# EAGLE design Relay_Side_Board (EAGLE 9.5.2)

## Sheet 1 of 2: Relay side expansion board for hoop house controller - main controller section
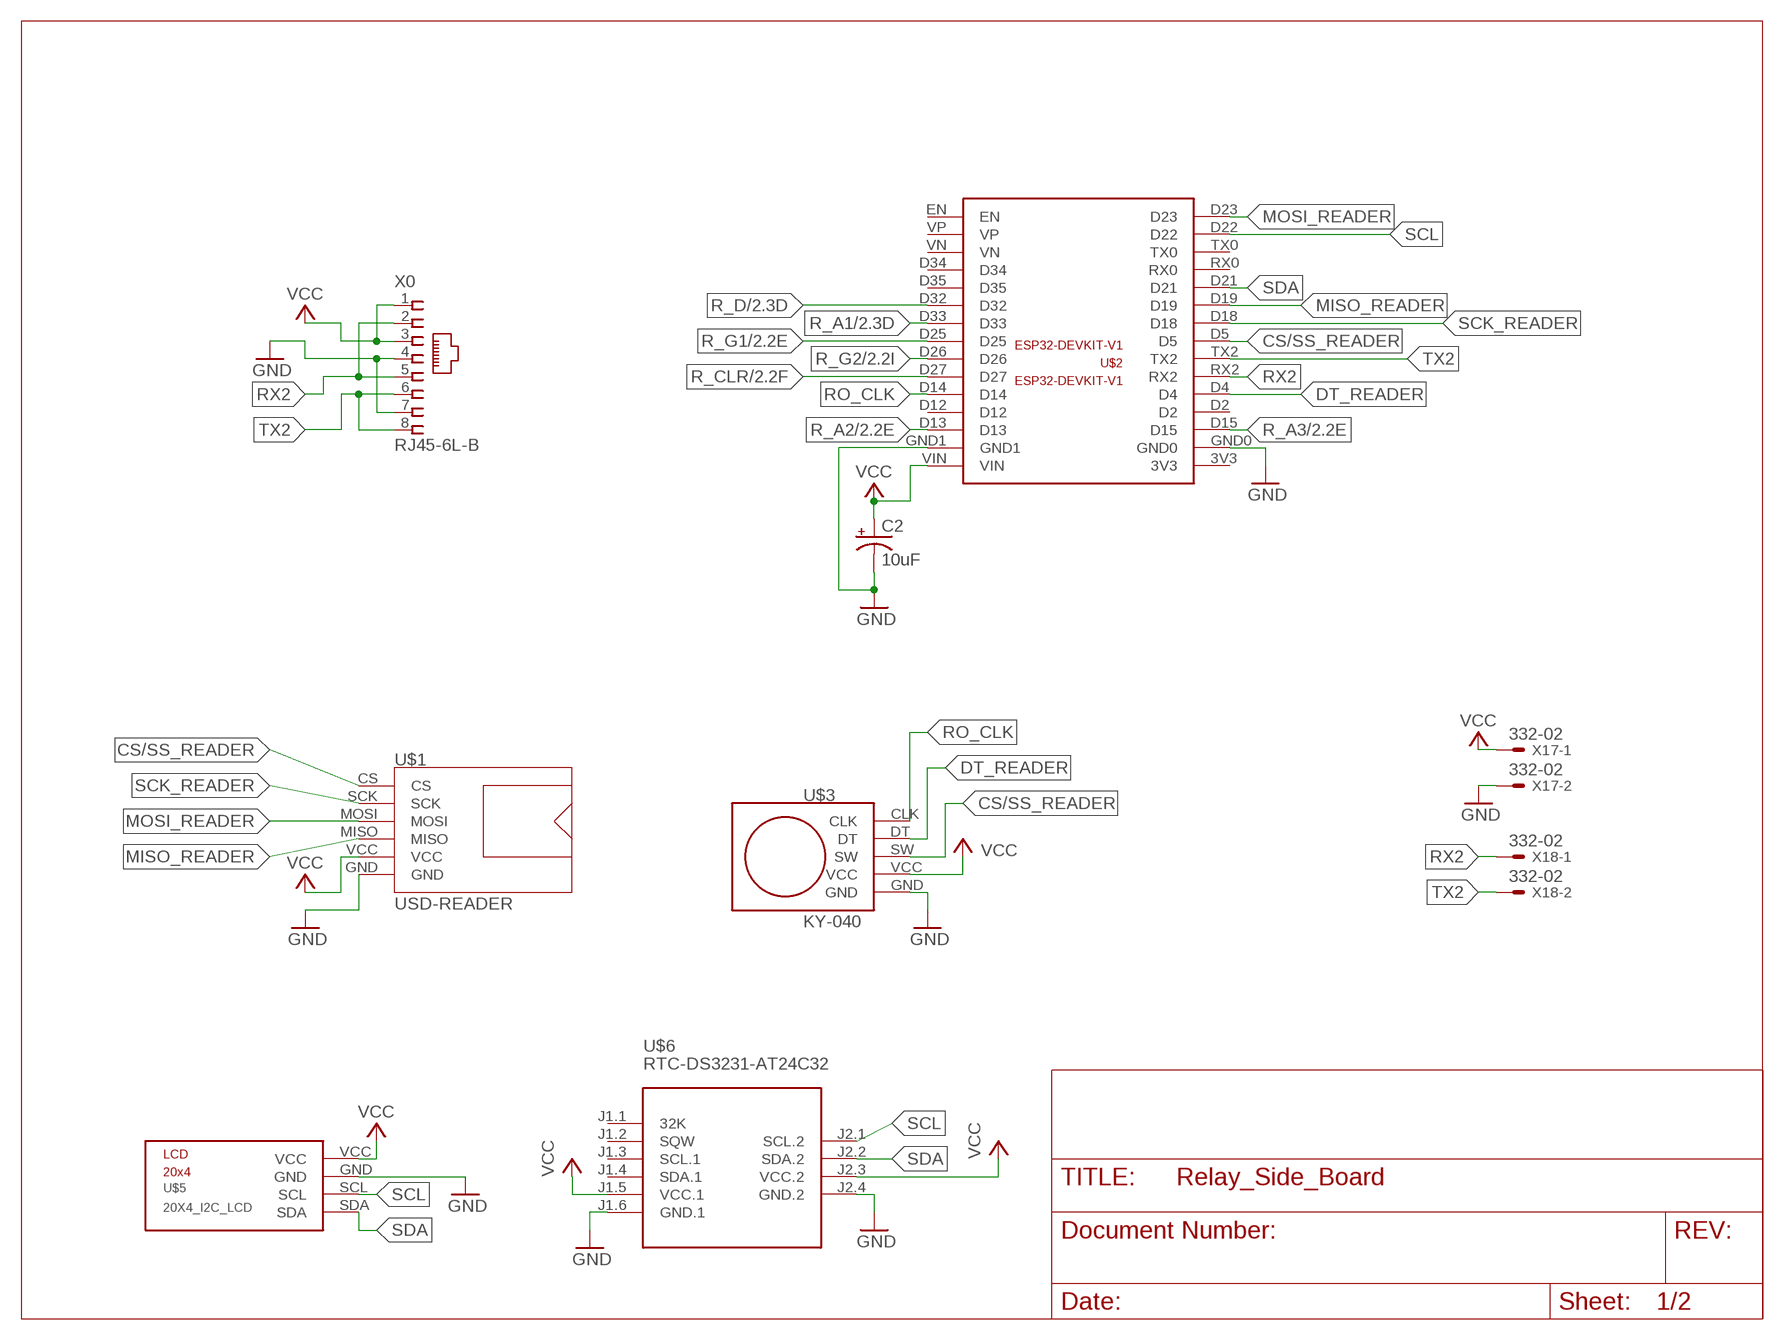
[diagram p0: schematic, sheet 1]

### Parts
C2  10uF  CPOL-USE3.5-10  [E3,5-10]
U$1  USD-READER  [USD-READER]
U$2  ESP32-DEVKIT-V1  [ESP32-DEVKIT-V1]
U$3  KY-040  [ROTARY-ENCODER]
U$5  20X4_I2C_LCD  [I2C_LCD]
U$6  RTC-DS3231-AT24C32  [RTC-DS3231-AT24C32]
X0  RJ45-6L-B  [RJ45-NO-SHIELD]
X17  332-02  [332-02]
X18  332-02  [332-02]

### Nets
CS/SS_READER: U$1.CS U$2.D5 U$3.SW
DT_READER: U$2.D4 U$3.DT
GND: C2.- U$1.GND U$2.GND0 U$2.GND1 U$3.GND U$5.GND U$6.J1.6(GND.1) U$6.J2.4(GND.2) X0.4 X0.7 X17.2 ; also sheet 2
MISO_READER: U$1.MISO U$2.D19
MOSI_READER: U$1.MOSI U$2.D23
R_A1: U$2.D33 ; also sheet 2
R_A2: U$2.D13 ; also sheet 2
R_A3: U$2.D15 ; also sheet 2
R_CLR: U$2.D27 ; also sheet 2
R_D: U$2.D32 ; also sheet 2
R_G1: U$2.D25 ; also sheet 2
R_G2: U$2.D26 ; also sheet 2
RO_CLK: U$2.D14 U$3.CLK
RX2: U$2.RX2 X0.2 X0.5 X18.1
SCK_READER: U$1.SCK U$2.D18
SCL: U$2.D22 U$5.SCL U$6.J2.1(SCL.2)
SDA: U$2.D21 U$5.SDA U$6.J2.2(SDA.2)
TX2: U$2.TX2 X0.6 X0.8 X18.2
VCC: C2.+ U$1.VCC U$2.VIN U$3.VCC U$5.VCC U$6.J1.5(VCC.1) U$6.J2.3(VCC.2) X0.1 X0.3 X17.1 ; also sheet 2
Unconnected: U$2.3V3 U$2.D2 U$2.D12 U$2.D34 U$2.D35 U$2.EN U$2.RX0 U$2.TX0 U$2.VN U$2.VP U$6.J1.1(32K) U$6.J1.2(SQW) U$6.J1.3(SCL.1) U$6.J1.4(SDA.1)

## Sheet 2 of 2: Relay side expansion board for hoop house controller - addressed relays with memory
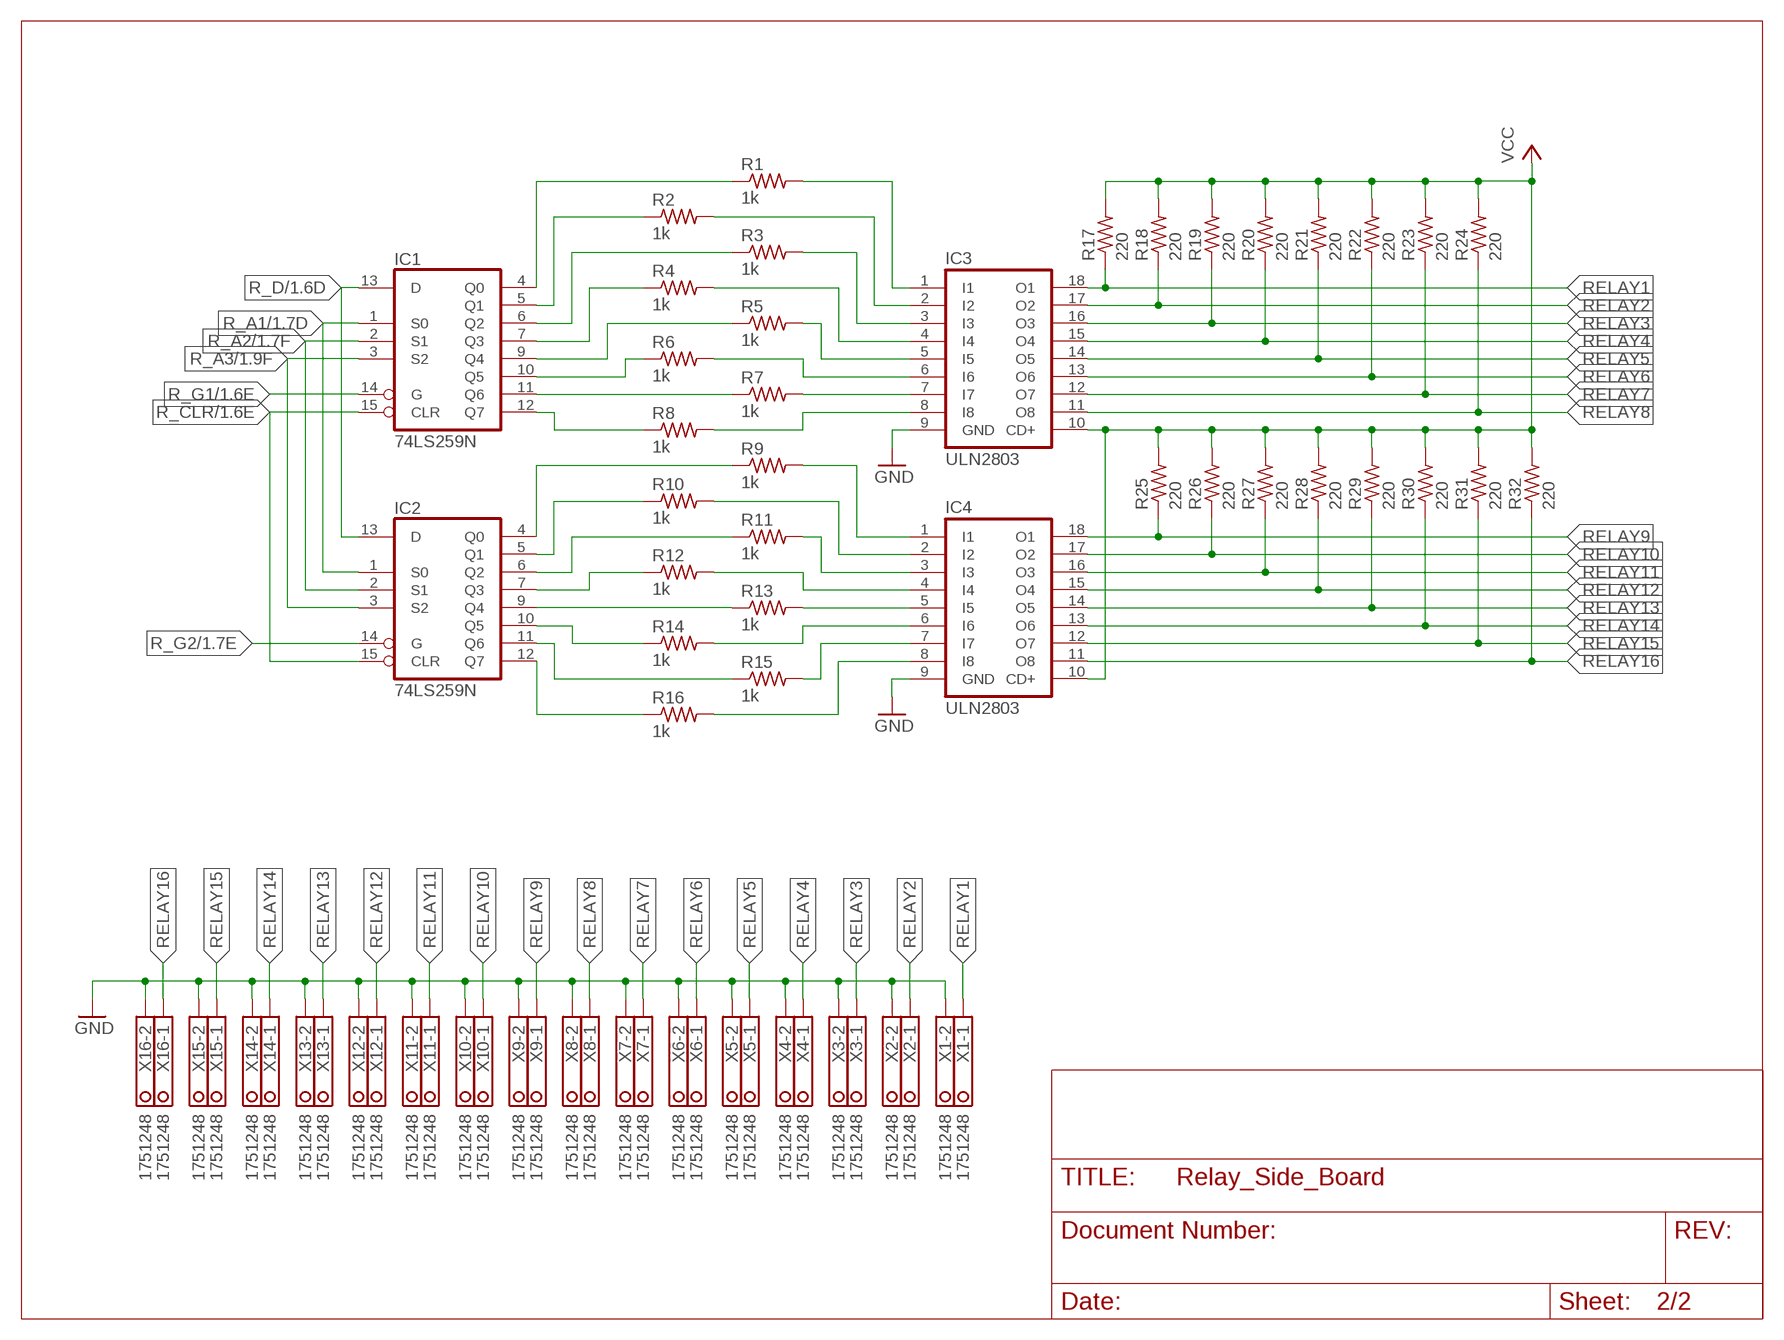
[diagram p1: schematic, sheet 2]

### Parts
IC1  74LS259N  [DIL16]
IC2  74LS259N  [DIL16]
IC3  ULN2803  ULN2803A  [DIL18]
IC4  ULN2803  ULN2803A  [DIL18]
R1  1k  R-US_R0805  [R0805]
R2  1k  R-US_R0805  [R0805]
R3  1k  R-US_R0805  [R0805]
R4  1k  R-US_R0805  [R0805]
R5  1k  R-US_R0805  [R0805]
R6  1k  R-US_R0805  [R0805]
R7  1k  R-US_R0805  [R0805]
R8  1k  R-US_R0805  [R0805]
R9  1k  R-US_R0805  [R0805]
R10  1k  R-US_R0805  [R0805]
R11  1k  R-US_R0805  [R0805]
R12  1k  R-US_R0805  [R0805]
R13  1k  R-US_R0805  [R0805]
R14  1k  R-US_R0805  [R0805]
R15  1k  R-US_R0805  [R0805]
R16  1k  R-US_R0805  [R0805]
R17  220  R-US_R0805  [R0805]
R18  220  R-US_R0805  [R0805]
R19  220  R-US_R0805  [R0805]
R20  220  R-US_R0805  [R0805]
R21  220  R-US_R0805  [R0805]
R22  220  R-US_R0805  [R0805]
R23  220  R-US_R0805  [R0805]
R24  220  R-US_R0805  [R0805]
R25  220  R-US_R0805  [R0805]
R26  220  R-US_R0805  [R0805]
R27  220  R-US_R0805  [R0805]
R28  220  R-US_R0805  [R0805]
R29  220  R-US_R0805  [R0805]
R30  220  R-US_R0805  [R0805]
R31  220  R-US_R0805  [R0805]
R32  220  R-US_R0805  [R0805]
X1  1751248  [1751248]
X2  1751248  [1751248]
X3  1751248  [1751248]
X4  1751248  [1751248]
X5  1751248  [1751248]
X6  1751248  [1751248]
X7  1751248  [1751248]
X8  1751248  [1751248]
X9  1751248  [1751248]
X10  1751248  [1751248]
X11  1751248  [1751248]
X12  1751248  [1751248]
X13  1751248  [1751248]
X14  1751248  [1751248]
X15  1751248  [1751248]
X16  1751248  [1751248]

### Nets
GND: IC3.9(GND) IC4.9(GND) X1.2 X2.2 X3.2 X4.2 X5.2 X6.2 X7.2 X8.2 X9.2 X10.2 X11.2 X12.2 X13.2 X14.2 X15.2 X16.2 ; also sheet 1
N$1: IC1.4(Q0) R1.1
N$2: IC1.5(Q1) R2.1
N$3: IC1.6(Q2) R3.1
N$4: IC1.7(Q3) R4.1
N$5: IC1.9(Q4) R5.1
N$6: IC1.10(Q5) R6.1
N$7: IC1.11(Q6) R7.1
N$8: IC1.12(Q7) R8.1
N$9: IC2.4(Q0) R9.1
N$10: IC2.5(Q1) R10.1
N$11: IC2.6(Q2) R11.1
N$12: IC2.7(Q3) R12.1
N$13: IC4.5(I5) R13.2
N$14: IC2.10(Q5) R14.1
N$15: IC2.11(Q6) R15.1
N$16: IC2.12(Q7) R16.1
N$17: IC3.1(I1) R1.2
N$18: IC3.2(I2) R2.2
N$19: IC3.3(I3) R3.2
N$20: IC3.4(I4) R4.2
N$21: IC3.5(I5) R5.2
N$22: IC3.6(I6) R6.2
N$23: IC3.7(I7) R7.2
N$24: IC3.8(I8) R8.2
N$25: IC2.9(Q4) R13.1
N$26: IC4.6(I6) R14.2
N$49: IC4.1(I1) R9.2
N$50: IC4.2(I2) R10.2
N$51: IC4.3(I3) R11.2
N$52: IC4.4(I4) R12.2
N$55: IC4.7(I7) R15.2
N$56: IC4.8(I8) R16.2
R_A1: IC1.1(S0) IC2.1(S0) ; also sheet 1
R_A2: IC1.2(S1) IC2.2(S1) ; also sheet 1
R_A3: IC1.3(S2) IC2.3(S2) ; also sheet 1
R_CLR: IC1.15(CLR) IC2.15(CLR) ; also sheet 1
R_D: IC1.13(D) IC2.13(D) ; also sheet 1
R_G1: IC1.14(G) ; also sheet 1
R_G2: IC2.14(G) ; also sheet 1
RELAY1: IC3.18(O1) R17.1 X1.1
RELAY2: IC3.17(O2) R18.1 X2.1
RELAY3: IC3.16(O3) R19.1 X3.1
RELAY4: IC3.15(O4) R20.1 X4.1
RELAY5: IC3.14(O5) R21.1 X5.1
RELAY6: IC3.13(O6) R22.1 X6.1
RELAY7: IC3.12(O7) R23.1 X7.1
RELAY8: IC3.11(O8) R24.1 X8.1
RELAY9: IC4.18(O1) R25.1 X9.1
RELAY10: IC4.17(O2) R26.1 X10.1
RELAY11: IC4.16(O3) R27.1 X11.1
RELAY12: IC4.15(O4) R28.1 X12.1
RELAY13: IC4.14(O5) R29.1 X13.1
RELAY14: IC4.13(O6) R30.1 X14.1
RELAY15: IC4.12(O7) R31.1 X15.1
RELAY16: IC4.11(O8) R32.1 X16.1
VCC: IC3.10(CD+) IC4.10(CD+) R17.2 R18.2 R19.2 R20.2 R21.2 R22.2 R23.2 R24.2 R25.2 R26.2 R27.2 R28.2 R29.2 R30.2 R31.2 R32.2 ; also sheet 1

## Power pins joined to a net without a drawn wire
GND: IC1.8(GND) IC2.8(GND)
VCC: IC1.16(VCC) IC2.16(VCC)

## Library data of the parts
C2 = rcl:CPOL-US: POLARIZED CAPACITOR, American symbol; SPICEPREFIX: C
IC1 IC2 = 74xx-us:74*259: 8-bit addressable LATCH
IC3 IC4 = uln-udn:ULN2803A: DRIVER ARRAY
R1-R32 = rcl:R-US_: RESISTOR, American symbol; SPICEPREFIX: R
U$1 = FF Hoop House Controller:USD-READER
U$2 = FF Hoop House Controller:ESP32-DEVKIT-V1
U$3 = FF Hoop House Controller:KY-040
U$5 = FF Hoop House Controller:20X4_I2C_LCD
U$6 = diy-modules:RTC-DS3231-AT24C32: RTC Module with Battery and EEPROM based on DS3231 and AT24C32 chips Tutorial can be found here: https://edwardmallon.wordpress.com/2014/05/21/using-a-cheap-3-ds3231-rtc-at24c32-eeprom-from-ebay/ Click here to find device on ebay.com
X0 = con-tycoelectronics:RJ45: CORCOM Modular RJ Jacks No Shield Source: www.tycoelectronics.com .. ENG_DS_1654001_1099_RJ_L_0507.pdf; MPN: RJ45-6L-B; OC_FARNELL: unknown; OC_NEWARK: 16R6090
X1-X16 = con-phoenix-350:1751248: MKDS 1/ 2-3,5 Printklemme; OC_FARNELL: unknown; OC_NEWARK: unknown
X17 X18 = con-garry:332-02: 2 Pin - 2mm Dual Row

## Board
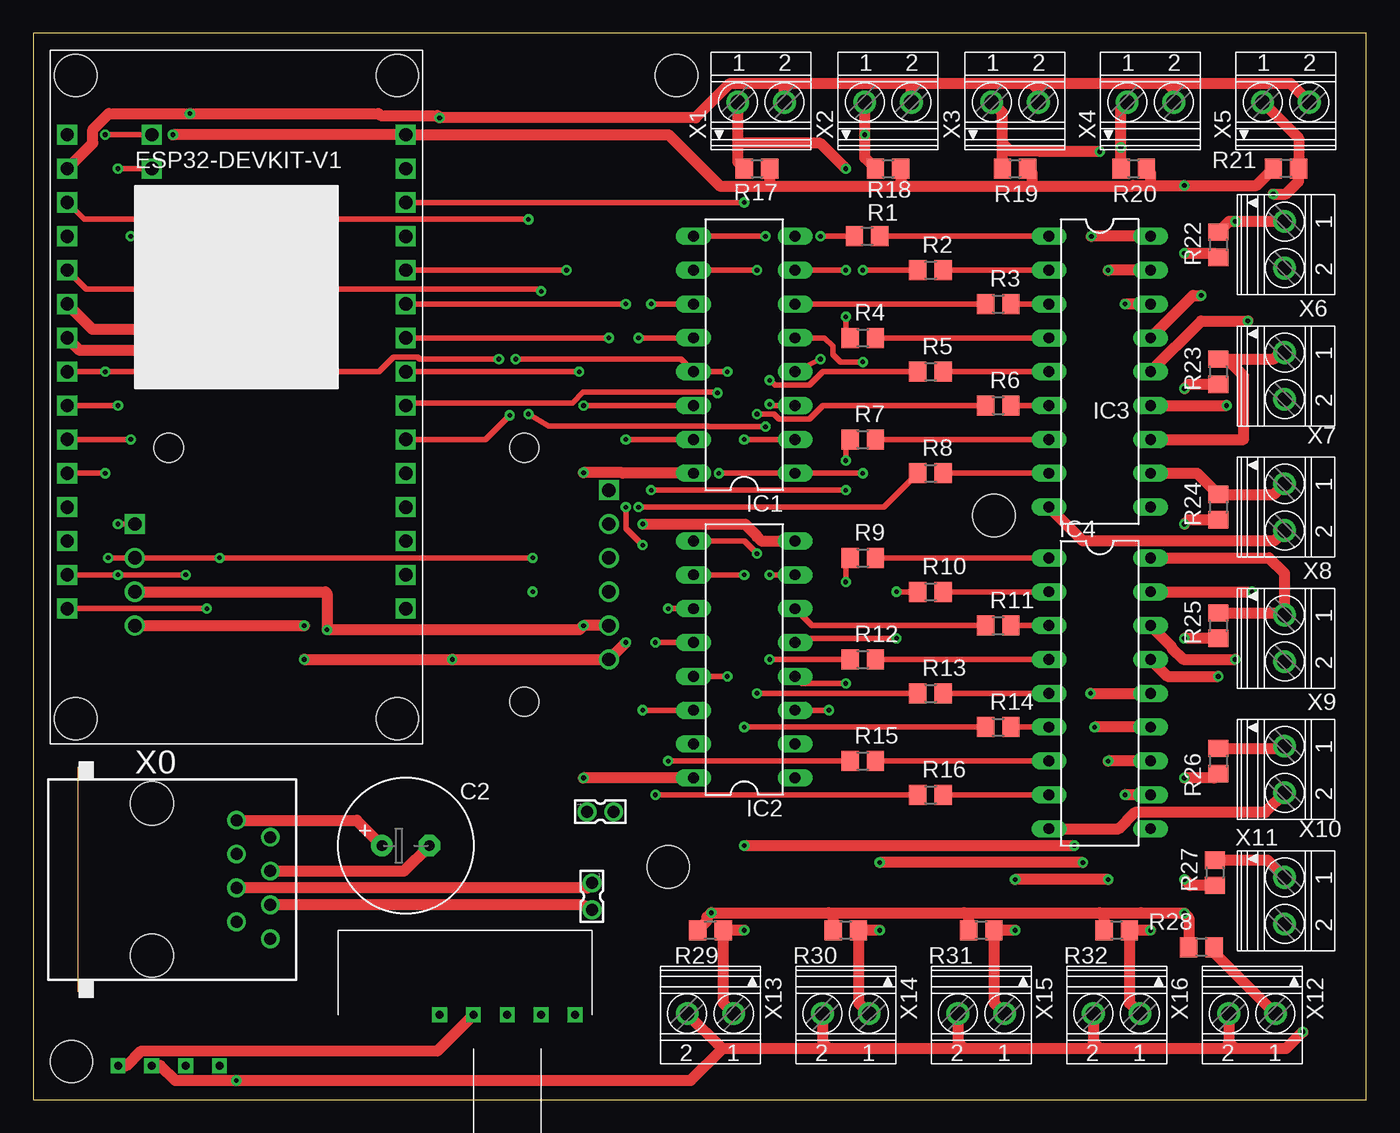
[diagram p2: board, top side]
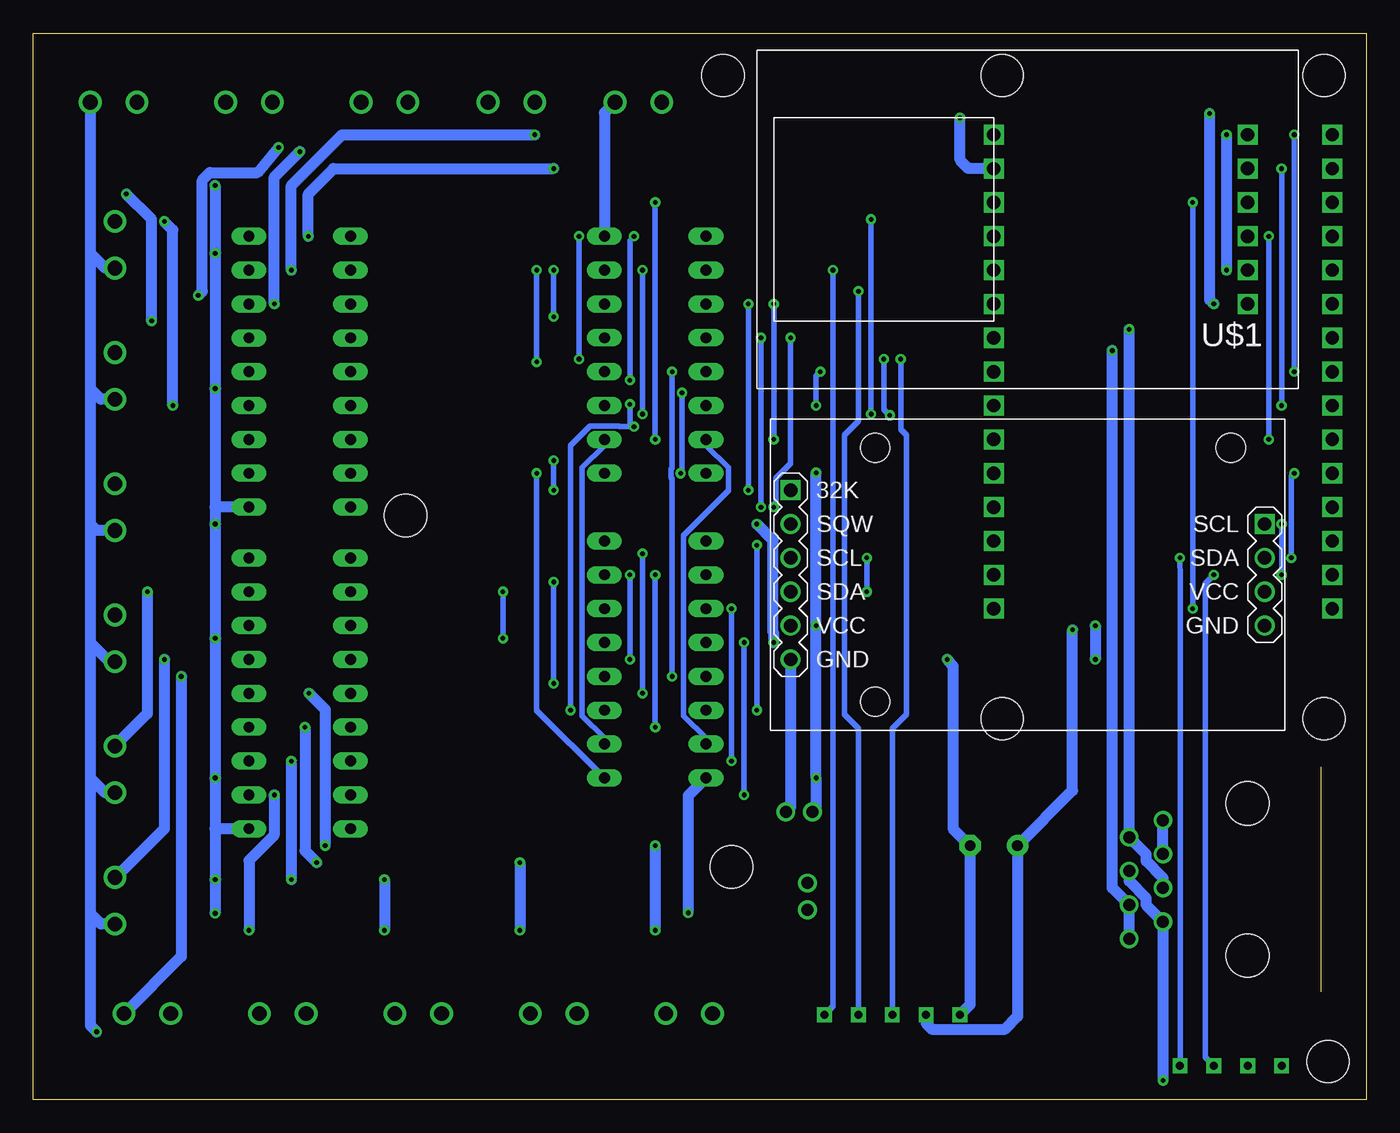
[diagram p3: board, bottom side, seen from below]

Size 100 x 80 mm. Coordinates in mm from the lower left corner, seen from the top.
Outline: 0,0 100,0 100,80 0,80 0,0
Copper layers (1*16): Top 0.035mm / dielectric 1.5mm / Bottom 0.035mm
Design rules "default": minimum track width 6mil, minimum drill 0.35mm, track to track 6mil, track to pad 6mil, pad to pad 6mil, via to via 6mil, smd to smd 6mil, copper to edge 40mil, drill to drill 6mil, minimum pad ring 10mil, minimum via ring 8mil, stop-mask expansion 4mil, vias tented up to drill 0mil, thermal gap 10mil
Holes 3.17 mm at 3.17,28.57 27.3,28.57 27.3,76.83 3.17,76.83 72.07,43.81 47.62,17.46 2.86,2.86 48.26,76.83

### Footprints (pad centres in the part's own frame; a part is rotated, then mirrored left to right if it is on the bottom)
E3,5-10 = drill 0.813 pad 1.6: + -1.778,0 | drill 0.813 pad 1.6 octagon: - 1.778,0
DIL16 = drill 0.813 long: 1 -8.89,-3.81; 2 -6.35,-3.81; 3 -3.81,-3.81; 4 -1.27,-3.81; 5 1.27,-3.81; 6 3.81,-3.81; 7 6.35,-3.81; 8 8.89,-3.81; 9 8.89,3.81; 10 6.35,3.81; 11 3.81,3.81; 12 1.27,3.81; 13 -1.27,3.81; 14 -3.81,3.81; 15 -6.35,3.81; 16 -8.89,3.81
DIL18 = drill 0.813 long: 1 -10.16,-3.81; 2 -7.62,-3.81; 3 -5.08,-3.81; 4 -2.54,-3.81; 5 0,-3.81; 6 2.54,-3.81; 7 5.08,-3.81; 8 7.62,-3.81; 9 10.16,-3.81; 10 10.16,3.81; 11 7.62,3.81; 12 5.08,3.81; 13 2.54,3.81; 14 0,3.81; 15 -2.54,3.81; 16 -5.08,3.81; 17 -7.62,3.81; 18 -10.16,3.81
R0805 = smd 1.3 x 1.5: 1 -0.95,0; 2 0.95,0
USD-READER = drill 1 square: CS -5.08,-6.35; GND -5.08,6.35; MISO -5.08,1.27; MOSI -5.08,-1.27; SCK -5.08,-3.81; VCC -5.08,3.81
ESP32-DEVKIT-V1 = drill 1 square: 3V3 -12.7,17.78; D2 -12.7,10.16; D4 -12.7,7.62; D5 -12.7,0; D12 12.7,10.16; D13 12.7,12.7; D14 12.7,7.62; D15 -12.7,12.7; D18 -12.7,-2.54; D19 -12.7,-5.08; D21 -12.7,-7.62; D22 -12.7,-15.24; D23 -12.7,-17.78; D25 12.7,0; D26 12.7,2.54; D27 12.7,5.08; D32 12.7,-5.08; D33 12.7,-2.54; D34 12.7,-10.16; D35 12.7,-7.62; EN 12.7,-17.78; GND0 -12.7,15.24; GND1 12.7,15.24; RX0 -12.7,-10.16; RX2 -12.7,5.08; TX0 -12.7,-12.7; TX2 -12.7,2.54; VIN 12.7,17.78; VN 12.7,-12.7; VP 12.7,-15.24
ROTARY-ENCODER = drill 0.6 square: CLK 0,5.08; DT 0,2.54; GND 0,-5.08; SW 0,0; VCC 0,-2.54
I2C_LCD = drill 0.6 square: GND 0,1.27; SCL 0,-1.27; SDA 0,-3.81; VCC 0,3.81
RTC-DS3231-AT24C32 = drill 1 square: J1.1 -17.78,6.35; J2.1 17.78,3.81 | drill 1: J1.2 -17.78,3.81; J1.3 -17.78,1.27; J1.4 -17.78,-1.27; J1.5 -17.78,-3.81; J1.6 -17.78,-6.35; J2.2 17.78,1.27; J2.3 17.78,-1.27; J2.4 17.78,-3.81 | hole 2.2: -11.43,-9.525; -11.43,9.525; 15.24,9.525
RJ45-NO-SHIELD = drill 0.9 pad 1.4: 1 -4.445,6.35; 2 -3.175,8.89; 3 -1.905,6.35; 4 -0.635,8.89; 5 0.635,6.35; 6 1.905,8.89; 7 3.175,6.35; 8 4.445,8.89 | hole 3.251: -5.715,0; 5.715,0
1751248 = drill 1.1 pad 1.7: 1 -1.75,-0.1; 2 1.75,-0.1
332-02 = drill 0.9 pad 1.27: 1 0,-1; 2 0,1

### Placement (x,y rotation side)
C2  27.94,19.05 0 top
IC1  53.34,55.88 90 top
IC2  53.34,33.02 90 top
IC3  80.01,54.61 270 top
IC4  80.01,30.48 270 top
R1  62.55,64.77 0 top
R2  67.31,62.23 0 top
R3  72.39,59.69 0 top
R4  62.23,57.15 0 top
R5  67.31,54.61 0 top
R6  72.39,52.07 0 top
R7  62.23,49.53 0 top
R8  67.31,46.99 0 top
R9  62.23,40.64 0 top
R10  67.31,38.1 0 top
R11  72.39,35.56 0 top
R12  62.23,33.02 0 top
R13  67.31,30.48 0 top
R14  72.39,27.94 0 top
R15  62.23,25.4 0 top
R16  67.31,22.86 0 top
R17  54.3,69.85 0 top
R18  64.14,69.85 0 top
R19  73.66,69.85 0 top
R20  82.55,69.85 0 top
R21  93.98,69.85 180 top
R22  88.9,64.14 270 top
R23  88.9,54.61 270 top
R24  88.9,44.45 270 top
R25  88.9,35.56 270 top
R26  88.9,25.4 270 top
R27  88.65,17.02 270 top
R28  87.63,11.43 180 top
R29  50.8,12.7 180 top
R30  60.96,12.7 180 top
R31  71.12,12.7 180 top
R32  81.28,12.7 180 top
U$1  13.97,66.04 180 bottom
U$2  15.24,54.61 0 top
U$3  35.56,6.35 270 top
U$5  10.16,2.54 90 top
U$6  25.4,39.37 0 bottom
X0  8.89,16.51 270 top
X1  54.61,74.93 0 top
X2  64.14,74.93 0 top
X3  73.66,74.93 0 top
X4  83.82,74.93 0 top
X5  93.98,74.93 0 top
X6  93.98,64.14 270 top
X7  93.98,54.29 270 top
X8  93.98,44.45 270 top
X9  93.98,34.61 270 top
X10  93.98,24.77 270 top
X11  93.98,14.92 270 top
X12  91.44,6.35 180 top
X13  50.8,6.35 180 top
X14  60.96,6.35 180 top
X15  71.12,6.35 180 top
X16  81.28,6.35 180 top
X17  42.55,21.59 270 top
X18  41.91,15.24 180 top

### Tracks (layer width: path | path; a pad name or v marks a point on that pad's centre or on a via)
CS/SS_READER  (via drill 0.35)
  Top 0.406: U$2.D5 v5.4,54.61 25.93,54.61 27.04,55.72 28.84,55.72 29,55.56 v34.92,55.56 | v5.4,72.39 U$1.CS
  Bottom 0.406: v5.4,72.39 v5.4,54.61 | U$3.SW 35.56,27.84 34.51,28.88 34.51,49.86 34.92,50.27 v34.92,55.56
DT_READER  (via drill 0.35)
  Top 0.406: v38.1,60.64 37.94,60.8 3.97,60.8 U$2.D4
  Bottom 0.406: v38.1,60.64 38.1,50.91 39.15,49.86 39.15,28.88 38.1,27.84 U$3.DT
GND  (via drill 0.35)
  Top 0.813: v11.43,59.69 U$1.GND | IC2.8 54.61,41.91 54.28,42.24 54.28,42.3 53.4,43.18 v45.72,43.18 | v44.45,34.29 U$6.J1.6 v31.43,33.02 v20.32,33.02 | U$6.J2.4 v20.32,35.56 | 56.52,76.24 52.28,76.24 49.7,73.66 v30.48,73.66 30.32,73.83 26.06,73.83 25.91,73.98 v11.75,73.98 5.66,73.98 4.46,72.78 4.46,71.77 U$2.GND0 | 56.52,76.24 66.04,76.24 | 66.04,76.24 74.93,76.24 | 74.93,76.24 85.09,76.24 | 85.09,76.24 94.32,76.24 X5.2 | v95.25,5.08 93.98,3.81 90.17,3.81 | 90.17,3.81 80.01,3.81 | 80.01,3.81 69.85,3.81 | 69.85,3.81 59.69,3.81 | 74.93,76.24 75.41,75.76 X3.2 | 85.09,76.24 85.57,75.76 X4.2 | 90.17,3.81 89.69,4.29 X12.2 | 80.01,3.81 79.53,4.29 X16.2 | 69.85,3.81 69.37,4.29 X15.2 | 59.69,3.81 59.21,4.29 X14.2 | 59.69,3.81 51.69,3.81 | IC3.9 78.74,41.91 93.09,41.91 X8.2 | IC4.9 81.44,20.32 82.66,21.54 92.4,21.54 X10.2 | 56.52,76.24 56.36,76.08 X1.2 | 66.04,76.24 65.89,76.08 X2.2 | U$5.GND 9.53,2.54 10.64,1.43 v15.24,1.43 49.31,1.43 51.69,3.81 | X13.2 51.69,3.81 | X0.4 27.81,17.14 C2.-
  Bottom 0.813: v11.43,59.69 11.75,60.01 v11.75,73.98 | v31.43,33.02 30.99,32.51 30.99,20.32 C2.- 29.72,7.11 U$3.GND | v44.45,34.29 44.45,34.97 44.49,35.02 44.49,41.95 v45.72,43.18 | v20.32,35.56 v20.32,33.02 | U$2.GND1 29.84,69.85 30.48,70.48 v30.48,73.66 | 95.73,63.5 95.73,53.34 | 95.73,53.34 95.73,43.18 | 95.73,43.18 95.73,34.29 | 95.73,34.29 95.73,24.13 | 95.73,24.13 95.73,13.97 | 95.73,13.97 95.73,5.56 v95.25,5.08 | 95.73,53.34 94.93,52.54 X7.2 | 95.73,43.18 95.25,42.7 X8.2 | 95.73,34.29 94.3,32.86 X9.2 | 95.73,24.13 94.61,23.02 X10.2 | 95.73,13.97 94.93,13.17 X11.2 | 95.73,63.5 94.61,62.38 X6.2 | IC1.8 57.15,74.04 X1.2 | X5.2 95.73,63.5 | X0.4 17.78,16.39 16.52,15.13 16.52,14.61 X0.7 v15.24,1.43 | U$6.J1.6 43.18,21.95 X17.2
MISO_READER  (via drill 0.35)
  Top 0.406: U$2.D19 v7.3,49.53 | v7.3,64.77 U$1.MISO
  Bottom 0.406: v7.3,49.53 v7.3,64.77
MOSI_READER  (via drill 0.35)
  Top 0.406: U$2.D23 v13.02,36.83 | v13.02,67.31 U$1.MOSI
  Bottom 0.406: v13.02,67.31 v13.02,36.83
N$1  (via drill 0.35)
  Top 0.406: IC1.4 v59.05,55.56 | R1.1 v59.05,64.77
  Bottom 0.406: v59.05,55.56 v59.05,64.77
N$2  (via drill 0.35)
  Top 0.406: R2.1 v62.23,62.23 | IC1.5 59.37,57.15 60.01,56.52 60.01,55.88 60.54,55.34 v62.23,55.34
  Bottom 0.406: v62.23,62.23 v62.23,55.34
N$3
  Top 0.406: R3.1 IC1.6
N$4  (via drill 0.35)
  Top 0.406: R4.1 60.96,57.47 v60.96,58.74 | v60.96,62.23 IC1.7
  Bottom 0.406: v60.96,58.74 v60.96,62.23
N$5  (via drill 0.35)
  Top 0.406: R5.1 59.25,54.61 58.23,53.59 55.63,53.59 v55.24,53.98 | v54.93,64.77 IC1.9
  Bottom 0.406: v54.93,64.77 55.24,64.45 v55.24,53.98
N$6  (via drill 0.35)
  Top 0.406: R6.1 59.25,52.07 58.23,51.05 55.94,51.05 55.56,51.44 v54.29,51.44 | v54.29,62.23 IC1.10
  Bottom 0.406: v54.29,62.23 v54.29,51.44
N$7  (via drill 0.35)
  Top 0.406: R7.1 60.96,49.21 v60.96,47.94 | v60.96,45.72 v46.35,45.72 | v46.35,59.69 IC1.11
  Bottom 0.406: v60.96,47.94 v60.96,45.72 | v46.35,59.69 v46.35,45.72
N$8  (via drill 0.35)
  Top 0.406: R8.1 63.82,44.45 v45.4,44.45 | v45.4,57.15 IC1.12
  Bottom 0.406: v45.4,57.15 v45.4,44.45
N$9  (via drill 0.35)
  Top 0.406: R9.1 60.96,40.32 v60.96,38.83 | v60.96,31.21 57.69,31.21 IC2.4
  Bottom 0.406: v60.96,38.83 v60.96,31.21
N$10  (via drill 0.35)
  Top 0.406: R10.1 v64.77,38.1 | v64.77,34.61 57.47,34.61 IC2.5
  Bottom 0.406: v64.77,38.1 v64.77,34.61
N$11
  Top 0.406: R11.1 58.42,35.56 IC2.6
N$12  (via drill 0.35)
  Top 0.406: R12.1 v55.24,33.02 | v55.24,39.37 IC2.7
  Bottom 0.406: v55.24,39.37 v55.24,33.02
N$13
  Top 0.406: R13.2 IC4.5
N$14  (via drill 0.35)
  Top 0.406: R14.1 v53.34,27.94 | v53.34,39.37 IC2.10
  Bottom 0.406: v53.34,39.37 v53.34,27.94
N$15  (via drill 0.35)
  Top 0.406: R15.1 v47.62,25.4 | v47.62,36.83 IC2.11
  Bottom 0.406: v47.62,36.83 v47.62,25.4
N$16  (via drill 0.35)
  Top 0.406: R16.1 v46.67,22.86 | v46.67,34.29 IC2.12
  Bottom 0.406: v46.67,22.86 v46.67,34.29
N$17
  Top 0.406: R1.2 IC3.1
N$18
  Top 0.406: R2.2 IC3.2
N$19
  Top 0.406: R3.2 IC3.3
N$20
  Top 0.406: R4.2 IC3.4
N$21
  Top 0.406: R5.2 IC3.5
N$22
  Top 0.406: R6.2 IC3.6
N$23
  Top 0.406: R7.2 IC3.7
N$24
  Top 0.406: R8.2 IC3.8
N$25  (via drill 0.35)
  Top 0.406: R13.1 v54.29,30.48 | v54.29,40.96 53.34,41.91 IC2.9
  Bottom 0.406: v54.29,30.48 v54.29,40.96
N$26
  Top 0.406: R14.2 IC4.6
N$49
  Top 0.406: R9.2 IC4.1
N$50
  Top 0.406: R10.2 IC4.2
N$51
  Top 0.406: R11.2 IC4.3
N$52
  Top 0.406: R12.2 IC4.4
N$55
  Top 0.406: R15.2 IC4.7
N$56
  Top 0.406: R16.2 IC4.8
R_A1  (via drill 0.35)
  Top 0.406: v51.34,53.02 51.27,53.09 41.25,53.09 40.44,52.27 28.14,52.27 U$2.D33 | v51.44,46.99 IC1.1 v62.23,46.99
  Bottom 0.406: v51.34,53.02 51.34,47.09 v51.44,46.99 | v62.23,46.99 62.23,29.21 IC2.1
R_A2  (via drill 0.35)
  Top 0.406: v53.34,49.53 IC1.2 | U$2.D13 v53.34,67.31
  Bottom 0.406: IC1.2 57.15,49.09 58.83,47.41 58.83,28.79 57.15,27.11 IC2.2 | v53.34,67.31 v53.34,49.53
R_A3  (via drill 0.35)
  Top 0.406: v54.93,50.48 50.67,50.48 50.61,50.55 38.67,50.55 v37.15,51.44 | IC1.3 55.34,52.07 v55.24,52.17 | v59.69,29.21 IC2.3 | v37.15,66.04 3.81,66.04 U$2.D15
  Bottom 0.406: v55.24,52.17 55.24,50.8 v54.93,50.48 56.01,50.48 56.07,50.55 58.23,50.55 59.69,49.09 v59.69,29.21 | v37.15,51.44 v37.15,66.04
R_CLR  (via drill 0.35)
  Top 0.406: U$2.D27 v44.45,59.69 | v44.45,49.53 IC1.15
  Bottom 0.406: v44.45,59.69 v44.45,49.53 | IC1.15 49.53,49.09 47.85,47.41 47.85,45.68 51.21,42.33 51.21,28.79 49.53,27.11 IC2.15
R_D  (via drill 0.35)
  Top 0.406: U$2.D32 33.94,49.53 v35.74,51.34 | v36.2,55.56 48.58,55.56 IC1.13 v52.07,54.61 | v52.07,31.75 IC2.13
  Bottom 0.406: v35.74,51.34 36.2,51.79 v36.2,55.56 | v52.07,54.61 52.07,47.39 52.17,47.29 52.17,46.69 52.07,46.59 v52.07,31.75
R_G1  (via drill 0.35)
  Top 0.406: U$2.D25 v40.96,54.61 | v41.27,52.07 IC1.14
  Bottom 0.406: v40.96,54.61 41.27,54.29 v41.27,52.07
R_G2  (via drill 0.35)
  Top 0.406: v44.45,44.45 44.45,42.86 v45.72,41.59 | U$2.D26 v43.18,57.15 | v45.72,29.21 IC2.14
  Bottom 0.406: v43.18,57.15 43.18,47.73 44.29,46.62 44.29,44.61 v44.45,44.45 | v45.72,41.59 v45.72,29.21
RELAY1  (via drill 0.35)
  Top 0.813: R17.1 52.86,70.33 52.86,71.75 | 52.86,71.75 X1.1 | IC3.18 v79.38,64.77 | v60.96,69.85 59.05,71.75 52.86,71.75
  Bottom 0.813: v79.38,64.77 79.38,67.94 77.47,69.85 v60.96,69.85
RELAY2  (via drill 0.35)
  Top 0.813: R18.1 62.38,70.65 v62.38,72.39 X2.1 | IC3.17 v80.64,62.23
  Bottom 0.813: v80.64,62.23 80.64,68.58 76.83,72.39 v62.38,72.39
RELAY3  (via drill 0.35)
  Top 0.813: R19.1 72.71,71.75 | 72.71,71.75 72.71,74.03 X3.1 | IC3.16 v81.92,59.69 | v80.01,71.12 75.53,71.12 75.49,71.16 73.31,71.16 72.71,71.75
  Bottom 0.813: v81.92,59.69 81.92,69.22 v80.01,71.12
RELAY4  (via drill 0.35)
  Top 0.813: R20.1 v81.6,71.44 81.6,74.36 X4.1 | IC3.15 87,60.33 v87.63,60.33
  Bottom 0.813: v87.63,60.33 87.33,60.63 87.33,68.98 86.76,69.55 83.17,69.55 v81.6,71.44
RELAY5  (via drill 0.35)
  Top 0.813: X5.1 94.93,72.13 R21.1 94.93,68.89 93.98,67.94 v93.03,67.94 | IC3.14 87.63,58.42 v91.12,58.42
  Bottom 0.813: v91.12,58.42 91.12,65.47 91.14,65.48 91.14,66.05 v93.03,67.94
RELAY6  (via drill 0.35)
  Top 0.813: R22.1 89.7,65.89 v90.17,65.89 X6.1 | IC3.13 v89.53,52.07
  Bottom 0.813: v89.53,52.07 89.53,65.25 v90.17,65.89
RELAY7
  Top 0.406: X7.1 93.75,56.17 93.69,56.17
  Top 0.813: R23.1 89.53,55.56 | 89.53,55.56 93.08,55.56 93.69,56.17 | IC3.12 90.81,49.53 90.81,54.29 89.53,55.56
RELAY8
  Top 0.813: X8.1 93.08,45.4 R24.1 87.31,46.99 IC3.11
RELAY9
  Top 0.813: R25.1 93.73,36.51 X9.1 93.88,39.47 92.71,40.64 IC4.18
RELAY10  (via drill 0.35)
  Top 0.813: R26.1 93.72,26.35 X10.1 | IC4.17 v91.44,38.1
  Bottom 0.813: v91.44,38.1 91.44,28.95 X10.1
RELAY11  (via drill 0.35)
  Top 0.813: R27.1 92.58,17.97 X11.1 | IC4.16 85.39,33.98 85.39,33.89 86.27,33.02 v90.17,33.02
  Bottom 0.813: v90.17,33.02 90.17,20.32 93.82,16.67 X11.1
RELAY12  (via drill 0.35)
  Top 0.813: X12.1 88.58,11.06 R28.1 | IC4.15 85.09,31.75 v88.9,31.75
  Bottom 0.813: v88.9,31.75 88.9,10.74 X12.1
RELAY13  (via drill 0.35)
  Top 0.813: X13.1 51.75,7.25 R29.1 v53.34,12.7 | v78.11,19.05 v53.34,19.05 | v79.32,30.48 IC4.14
  Bottom 0.813: v53.34,19.05 v53.34,12.7 | v79.32,30.48 78.11,29.26 v78.11,19.05
RELAY14  (via drill 0.35)
  Top 0.813: X14.1 61.91,7.25 R30.1 v63.5,12.7 | IC4.13 v79.62,27.94 | v78.74,17.78 v63.5,17.78
  Bottom 0.813: v79.62,27.94 79.62,18.66 v78.74,17.78 | v63.5,17.78 v63.5,12.7
RELAY15  (via drill 0.35)
  Top 0.813: X15.1 72.07,7.25 R31.1 v73.66,12.7 | IC4.12 v80.64,25.4 | v80.64,16.51 v73.66,16.51
  Bottom 0.813: v80.64,25.4 v80.64,16.51 | v73.66,16.51 v73.66,12.7
RELAY16  (via drill 0.35)
  Top 0.813: X16.1 82.23,7.25 R32.1 v83.82,12.7 | IC4.11 v81.92,22.86
  Bottom 0.813: v81.92,22.86 81.94,22.84 81.94,19.82 83.82,17.93 v83.82,12.7
RO_CLK  (via drill 0.35)
  Top 0.406: U$2.D14 v40.01,62.23
  Bottom 0.406: v40.01,62.23 40.01,6.99 U$3.CLK
RX2  (via drill 0.35)
  Top 0.813: v17.78,57.78 4.45,57.78 U$2.RX2 | X18.1 41.55,15.88 X0.5
  Bottom 0.813: X0.5 15.24,16.63 16.5,17.89 16.5,18.41 X0.2 v17.78,57.78
SCK_READER  (via drill 0.35)
  Top 0.406: U$2.D18 v6.35,52.07 | v6.35,69.85 U$1.SCK
  Bottom 0.406: v6.35,69.85 v6.35,52.07
SCL  (via drill 0.35)
  Top 0.406: U$6.J2.1 v6.35,43.18 | U$2.D22 v6.35,39.37 v11.43,39.37
  Bottom 0.406: v6.35,43.18 v6.35,39.37 | U$5.SCL 12.06,3.17 12.06,38.73 v11.43,39.37
SDA  (via drill 0.35)
  Top 0.406: v37.47,40.64 v13.97,40.64 U$6.J2.2 v5.62,40.64 | U$2.D21 v5.4,46.99
  Bottom 0.406: v37.47,40.64 v37.47,38.1 | v5.4,46.99 5.62,46.77 v5.62,40.64 | U$5.SDA 13.96,2.55 13.96,39.04 v13.97,40.64
TX2  (via drill 0.35)
  Top 0.813: v19.05,56.2 3.49,56.2 U$2.TX2 | X0.6 41.27,14.61 41.64,14.24 X18.2
  Bottom 0.813: X0.8 X0.6 19.05,15.88 v19.05,56.2
VCC  (via drill 0.35)
  Top 0.813: v10.48,72.39 U$2.VIN 47.66,72.39 51.51,68.54 55.24,68.54 | v10.48,62.23 U$1.VCC | U$6.J2.3 21.91,38.1 22.04,37.97 v22.04,35.24 40.96,35.24 v41.27,35.56 U$6.J1.5 | IC1.16 44.21,46.99 44.16,47.03 v41.27,47.03 | 83.82,68.58 82.52,68.58 82.48,68.54 74.93,68.54 | 83.82,68.58 v86.36,68.58 91.76,68.58 R21.2 | 55.24,68.54 65.41,68.54 | 65.41,68.54 74.93,68.54 | R28.2 86.68,13.65 v86.36,13.97 83.15,13.97 83.11,14.01 80.01,14.01 | R27.2 86.8,16.07 v86.36,16.51 | R26.2 88.58,24.13 v86.36,24.13 | R25.2 v86.36,34.61 | R24.2 86.68,43.5 v86.36,43.18 | R20.2 83.82,69.53 83.82,68.58 | R19.2 74.93,69.53 74.93,68.54 | R29.2 50.54,13.39 50.54,13.68 v50.87,14.01 59.69,14.01 | 59.69,14.01 69.85,14.01 | 69.85,14.01 80.01,14.01 | 59.69,14.01 60.01,13.69 R30.2 | 69.85,14.01 70.17,13.69 R31.2 | 80.01,14.01 80.33,13.69 R32.2 | v86.36,63.5 88.58,63.5 R22.2 | R17.2 55.24,68.54 | R18.2 65.08,68.86 65.41,68.54 | U$5.VCC 6.99,2.54 8.11,3.65 30.32,3.65 U$3.VCC | IC2.16 v41.27,24.13 | R23.2 86.68,53.66 v86.36,53.34 | X0.1 24.26,20.95 C2.+
  Bottom 0.813: v10.48,72.39 v10.48,62.23 | v86.36,68.58 v86.36,63.5 v86.36,53.34 86.36,44.45 | 86.36,44.45 v86.36,43.18 v86.36,34.61 v86.36,24.13 86.36,20.32 | 86.36,20.32 v86.36,16.51 v86.36,13.97 | IC3.10 86.36,44.45 | IC4.10 86.36,20.32 | IC2.16 50.87,22.79 v50.87,14.01 | U$3.VCC 33.02,5.72 32.53,5.24 27.16,5.24 26.16,6.23 C2.+ 22.04,23.18 v22.04,35.24 | v41.27,47.03 v41.27,35.56 v41.27,24.13 41.27,21.86 X17.1 | X0.3 X0.1

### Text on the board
tValues: 2020 Winter - V0 / University of Washington / EE Capstone / Relay Board | ~ - | ~ - | ~ - | ~ - | ~ - | - ~ | - ~ | - ~ | - ~ | - ~ | + - | - ~ | RX / / TX | - + SW DT CLK | + - SCL SDA | - ~ | - ~ | - ~ | - ~ | - ~

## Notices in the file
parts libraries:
diy-modules: Released under the Creative Commons Attribution 4.0 International License: http://creativecommons.org/licenses/by/4.0
